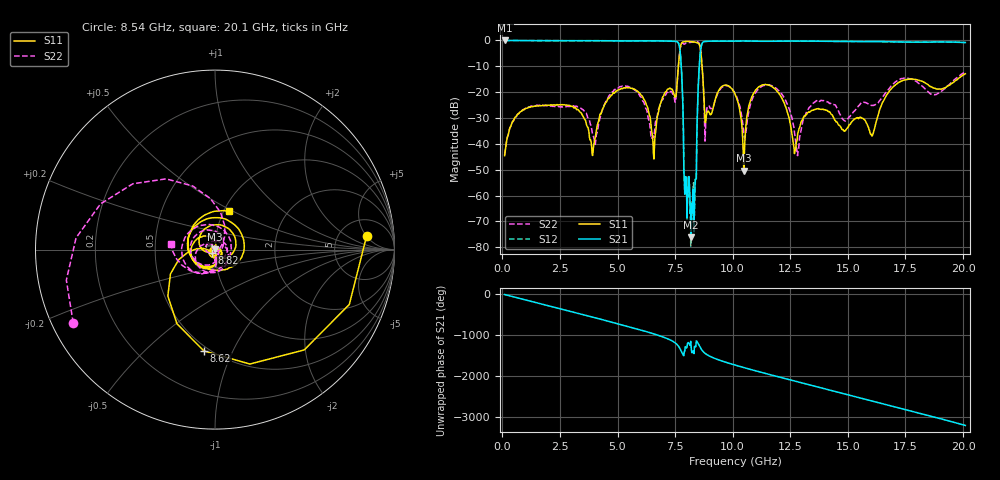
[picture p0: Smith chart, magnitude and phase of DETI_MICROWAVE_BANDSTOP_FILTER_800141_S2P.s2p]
! 4/18/2019 1:47:01 PM
! CHANNEL.2
! TR.MEASUREMENT
! CORRECTED.DATA
# GHZ S RI R 50.0
! FREQ.GHZ  S11RE  S11IM  S21RE  S21IM  S12RE  S12IM  S22RE  S22IM
!; PortSelection: Port_12
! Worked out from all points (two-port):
!   1001 points, 100 MHz to 20.1 GHz, reference 50 ohm
!   highest |S21| = -0.03 dB at 120 MHz (marker M1); lowest = -76.1 dB at 8.2 GHz (marker M2)
!   |S21| within 3 dB of the highest: start of sweep to 7.7 GHz; 8.62 GHz to end of sweep
!   lowest |S11| = -50.4 dB at 10.48 GHz (marker M3), VSWR 1.01, Z = 49.8 + j0.256 ohm
!   |S11| at or under -10 dB: start of sweep to 7.642 GHz; 8.672 GHz to end of sweep
!   |S22| runs from -44.5 to -0.5 dB; largest |S21 - S12| = 0.014
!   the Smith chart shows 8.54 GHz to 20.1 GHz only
!   S11 on the Smith chart (normalised r, x): 8.54 GHz: 9, +5; 8.62 GHz: 0.47, -0.78; 8.82 GHz: 0.97, -0.04; 20.1 GHz: 1.06, +0.48
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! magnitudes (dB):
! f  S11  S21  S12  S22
! 100 MHz  -44.6  0.0  0.0  -44.3
! 120 MHz  -43.2  0.0  0.0  -43.0
! 1.04 GHz  -26.3  -0.1  -0.1  -26.2
! 3.44 GHz  -28.3  -0.1  -0.1  -26.4
! 3.92 GHz  -44.5  -0.1  -0.1  -36.3
! 5.06 GHz  -19.0  -0.2  -0.2  -18.1
! 6.78 GHz  -27.7  -0.2  -0.2  -26.6
! 7.66 GHz  -8.2  -1.4  -1.4  -8.2
! 7.96 GHz  -0.4  -52.7  -52.8  -1.0
! 8.2 GHz  -0.5  -76.1  -62.5  -0.7
! 8.34 GHz  -0.6  -62.1  -67.7  -0.5
! 8.54 GHz  -1.4  -11.3  -11.3  -1.0
! 8.62 GHz  -4.9  -3.0  -3.0  -4.6
! 8.82 GHz  -31.8  -0.4  -0.4  -33.6
! 10.1 GHz  -20.7  -0.3  -0.2  -20.4
! 10.48 GHz  -50.4  -0.2  -0.2  -35.9
! 11.24 GHz  -17.4  -0.3  -0.3  -17.9
! 12.8 GHz  -38.3  -0.2  -0.2  -44.3
! 13.44 GHz  -27.0  -0.3  -0.3  -24.7
! 16.04 GHz  -37.0  -0.4  -0.4  -25.1
! 16.78 GHz  -19.9  -0.5  -0.5  -18.7
! 20.1 GHz  -12.9  -0.8  -0.8  -12.2
